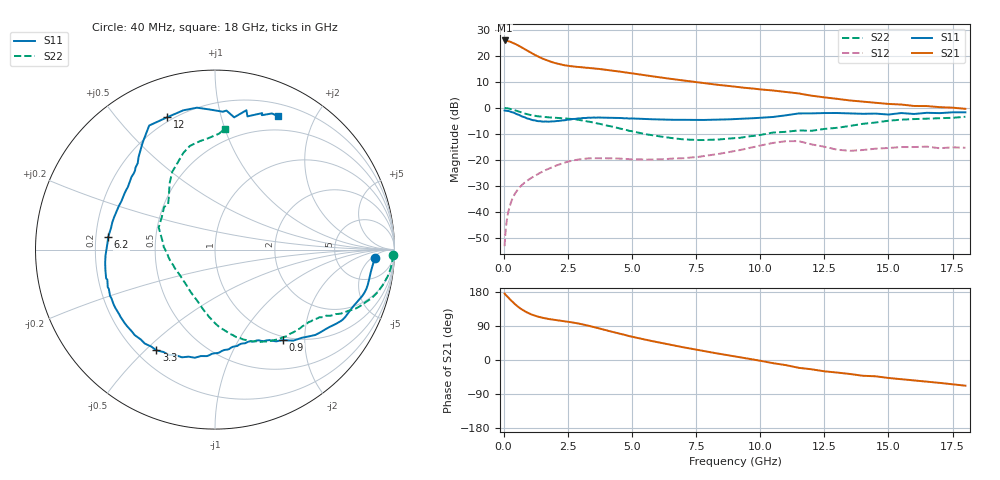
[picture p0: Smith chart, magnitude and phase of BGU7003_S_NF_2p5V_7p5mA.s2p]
!	Filename:	P:\Prog\Test\Noise\ATS_data\Testdata_Net\BGU7002	BGU7003	RN20082092\BGU7003_B1_high	freq_bias	loop_2.53V6.82mA_D.s2p
!	Date/Time:	Tue	16-Sep-08	9:22:46
!	BGU7003_B1_high	freq_bias	loop
!	bias	mode	1:00	Vout=	2.53	"V,"	Iout=	6.955	"mA,"	Vin=	3.283	"V,"	Iin=	0.71	mA
!	Date/time	Sun	Aug	10	23:33:24	2008
!	Device	data	file	deembeded	for	feedlines	and	parallel
!	Original	file:	\BGU7002	BGU7003	RN20082092\BGU7003_B1_high	freq_bias	loop_2.53V6.82mA_R.s2p
!	Feed-files:	PR029V01_high	"frequency_140808_Feed1.s2p,"	PR029V01_high	frequency_140808_Feed2.s2p
!	Parallel-file:	PR029V01_high	frequency_140808_Par.s2p
#	MHz	S	MA	R	50
!	Freq-MHz	S11-mag	S11-arg	S21-mag	S21-arg	S12-mag	S12-arg	S22-mag	S22-arg
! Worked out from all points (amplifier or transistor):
!   152 points, 40 MHz to 18 GHz, reference 50 ohm
!   highest |S21| = 25.8 dB at 40 MHz (marker M1)
!   |S21| within 3 dB of that: start of sweep to 760.3 MHz
!   unconditionally stable (mu >= 1): nowhere
!   at 290 MHz: K = 0.21, MSG = 30.7 dB, |S12| = -36.1 dB
!   at 2.05 GHz: K = 0.56, MSG = 19.6 dB, |S12| = -22.1 dB
!   at 18 GHz: K = 0.67, MSG = 7.5 dB, |S12| = -15.3 dB
!   lowest NFmin = 0.50 dB at 400 MHz
!   S11 on the Smith chart (normalised r, x): 40 MHz: 14, -6; 900 MHz: 0.94, -1.58; 3.3 GHz: 0.28, -0.54; 6.2 GHz: 0.25, +0.06; 12 GHz: 0.18, +0.69; 18 GHz: 0.33, +1.52
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40  0.8905 -3.0  19.52 175.3  0.00225 78.0  0.9936 -1.7
140  0.8747 -10.8  19.15 168.2  0.00777 81.8  0.983 -6.5
240  0.8557 -18.2  18.58 160.8  0.01309 78.6  0.9617 -10.8
440  0.7913 -31.5  16.93 147.7  0.02266 72.5  0.9007 -18.3
550  0.7469 -38.0  15.82 141.3  0.0272 69.9  0.8655 -21.5
650  0.7131 -42.7  14.88 136.1  0.03105 67.7  0.8309 -23.9
900  0.6315 -53.0  12.59 126.0  0.03963 64.0  0.7614 -28.2
1100  0.5877 -59.1  11.08 119.8  0.04617 62.0  0.7211 -30.7
1250  0.5717 -62.9  10.15 116.2  0.05128 60.5  0.7002 -32.6
1650  0.5482 -72.3  8.273 109.5  0.06488 56.7  0.6641 -37.2
1950  0.5503 -79.5  7.338 106.1  0.0751 53.0  0.6479 -41.2
2350  0.5772 -90.0  6.578 102.5  0.08834 46.9  0.6288 -48.1
3100  0.6403 -113.6  5.955 93.7  0.1058 33.3  0.5726 -64.1
3300  0.6494 -120.2  5.835 90.6  0.1079 29.8  0.5503 -68.4
4700  0.6306 -159.8  4.802 66.4  0.1055 15.5  0.3832 -93.8
6200  0.599 173.2  3.767 44.2  0.1039 15.7  0.2794 -116.8
7400  0.5881 157.1  3.149 28.6  0.113 17.7  0.2435 -139.6
9200  0.6166 139.0  2.487 7.3  0.1552 17.5  0.2665 -175.1
12000  0.7841 109.8  1.71 -24.5  0.2 -27.8  0.3636 135.9
12500  0.7958 102.8  1.589 -29.8  0.1805 -31.9  0.3947 130.5
15500  0.796 77.3  1.159 -50.6  0.1776 -33.6  0.5944 103.6
18000  0.822 64.9  0.9582 -67.8  0.1721 -46.7  0.6752 85.4
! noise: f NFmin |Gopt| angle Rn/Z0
400  0.498  0.307  9.15  0.13
1000  0.609  0.301  24.76  0.144
1500  0.701  0.299  37.77  0.15
1700  0.737  0.298  42.97  0.151
2200  0.829  0.297  55.99  0.15
3000  0.976  0.298  76.8  0.143
4400  1.234  0.308  113.2  0.117
5800  1.491  0.328  149.7  0.09
8000  1.896  0.381  -160.3  0.087
1.2e+04  2.632  0.542  -121.9  0.392
